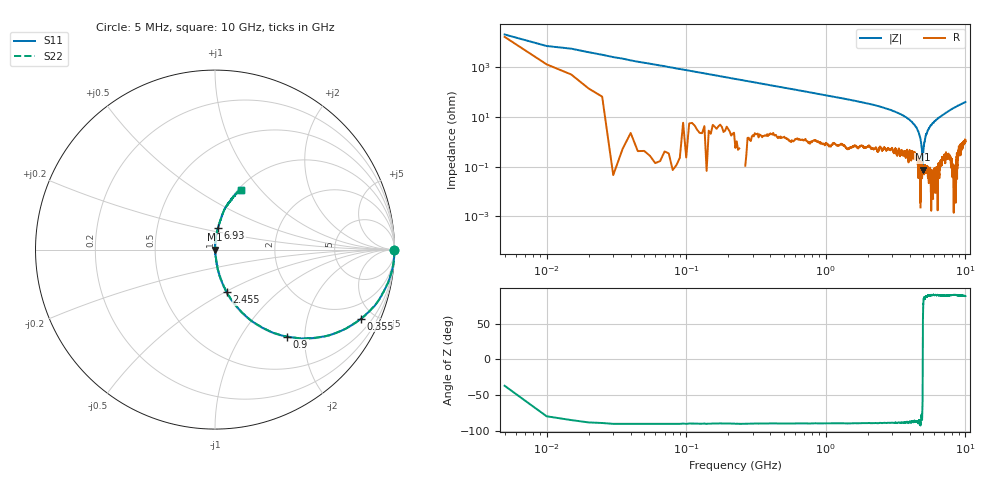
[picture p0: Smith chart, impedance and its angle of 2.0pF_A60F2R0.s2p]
! Amotech Co.,Ltd.
! http://www.amotech.co.kr/
! Part Number: A60F2R0
! These Parameters are Measured in Series Mode Connection
! Operation Temp=25[degC], DC Bias Voltage=0[V]
! Freq. Start=5[MHz] Stop=10[GHz], 2000[Steps]
! Date: Monday, July 20, 2020, 03:18:37
# GHZ S RI R 50.000000
!Freq.(Hz) S11(Real) S11(Imag) S21(Real) S21(Imag) S12(Real) S12(Imag) S22(Real) S22(Imag)
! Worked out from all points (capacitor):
!   2000 points, 5 MHz to 10 GHz, reference 50 ohm
!   read as one part in series: C = 2.12 pF near 55 MHz
!   lowest |Z| = 75.6 mohm at 4.945 GHz (marker M1)
!   series resonance near 4.944 GHz, so ESL is about 490 pH
!   S11 on the Smith chart (normalised r, x): 5 MHz: open; 355 MHz: 1.03, -4.22; 900 MHz: 1.02, -1.64; 2.455 GHz: 1.01, -0.51; 6.93 GHz: 1.00, +0.25; 10 GHz: 1.02, +0.79
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0.005  0.9961 -0.00293  0.00393 0.00293  0.00393 0.00293  0.9961 -0.00293
0.06  0.9936 -0.0795  0.00637 0.0795  0.00637 0.0795  0.9936 -0.0795
0.105  0.9799 -0.1367  0.0201 0.1367  0.0201 0.1367  0.9799 -0.1367
0.205  0.9293 -0.2528  0.0707 0.2528  0.0707 0.2528  0.9293 -0.2528
0.355  0.8143 -0.3848  0.1857 0.3848  0.1857 0.3848  0.8143 -0.3848
0.9  0.4019 -0.4843  0.5981 0.4843  0.5981 0.4843  0.4019 -0.4843
1.675  0.1551 -0.3551  0.8449 0.3551  0.8449 0.3551  0.1551 -0.3551
2.455  0.0669 -0.2377  0.9331 0.2377  0.9331 0.2377  0.0669 -0.2377
3.34  0.0235 -0.133  0.9765 0.133  0.9765 0.133  0.0235 -0.133
3.955  0.00926 -0.078  0.9907 0.078  0.9907 0.078  0.00926 -0.078
4.495  0.00345 -0.0339  0.9966 0.0339  0.9966 0.0339  0.00345 -0.0339
4.78  0.000293 -0.0121  0.9997 0.0121  0.9997 0.0121  0.000293 -0.0121
4.945  0.000727 0.000205  0.9993 -0.000205  0.9993 -0.000205  0.000727 0.000205
5.005  0.000884 0.0045  0.9991 -0.0045  0.9991 -0.0045  0.000884 0.0045
5.065  0.00056 0.00844  0.9994 -0.00844  0.9994 -0.00844  0.00056 0.00844
5.175  0.000943 0.0153  0.9991 -0.0153  0.9991 -0.0153  0.000943 0.0153
5.41  0.00142 0.0308  0.9986 -0.0308  0.9986 -0.0308  0.00142 0.0308
5.825  0.00351 0.0568  0.9965 -0.0568  0.9965 -0.0568  0.00351 0.0568
6.67  0.0126 0.1045  0.9874 -0.1045  0.9874 -0.1045  0.0126 0.1045
6.93  0.0172 0.1207  0.9828 -0.1207  0.9828 -0.1207  0.0172 0.1207
8.335  0.0533 0.2238  0.9467 -0.2238  0.9467 -0.2238  0.0533 0.2238
10  0.1421 0.3347  0.8579 -0.3347  0.8579 -0.3347  0.1421 0.3347
